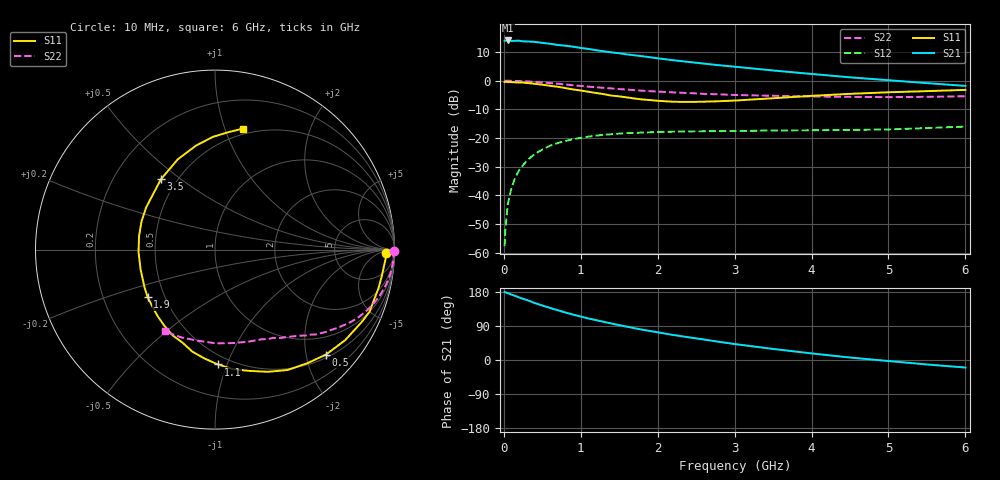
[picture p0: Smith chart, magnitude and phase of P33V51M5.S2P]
! SIEMENS Small Signal Semiconductors
! BFP181
! Si NPN RF Bipolar Junction Transistor in SOT143
! VCE = 3.5 V  IC = 1.5 mA
! Common Emitter S-Parameters:  March  1996
# GHz  S  MA  R  50
!  f  S11  S21  S12  S22
! GHz  MAG  ANG  MAG  ANG  MAG  ANG  MAG  ANG
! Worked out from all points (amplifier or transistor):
!   36 points, 10 MHz to 6 GHz, reference 50 ohm
!   highest |S21| = 14.0 dB at 50 MHz (marker M1)
!   |S21| within 3 dB of that: start of sweep to 1.109 GHz
!   unconditionally stable (mu >= 1): 2.733 GHz to end of sweep
!   at 250 MHz: K = 0.10, MSG = 21.6 dB, |S12| = -29.4 dB
!   at 1.4 GHz: K = 0.57, MSG = 14.3 dB, |S12| = -18.7 dB
!   at 6 GHz: K = 1.20, MAG = 4.4 dB, |S12| = -16.0 dB
!   S11 on the Smith chart (normalised r, x): 10 MHz: 36, -13; 500 MHz: 0.57, -2.40; 1.1 GHz: 0.43, -0.93; 1.9 GHz: 0.40, -0.27; 3.5 GHz: 0.41, +0.42; 6 GHz: 0.45, +1.15
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0.01  0.9514 -1.0  4.977 179.5  0.0013 81.9  0.9982 -0.3
0.02  0.9545 -2.0  4.986 179.0  0.0025 89.8  0.9978 -0.8
0.05  0.9488 -4.3  5.03 176.3  0.0069 91.1  0.9951 -2.0
0.1  0.941 -9.0  4.934 172.7  0.0136 82.5  0.9943 -4.1
0.2  0.9292 -17.6  4.968 165.0  0.0275 79.3  0.9856 -8.1
0.4  0.8836 -34.8  4.758 150.5  0.0526 68.3  0.9532 -15.7
0.5  0.8511 -43.4  4.569 143.6  0.0629 63.2  0.9317 -19.1
0.6  0.8158 -50.9  4.405 137.5  0.0732 58.3  0.9083 -22.3
0.8  0.7425 -66.5  4.073 125.3  0.0889 50.5  0.8599 -27.8
0.9  0.7037 -73.9  3.916 119.8  0.0955 46.6  0.8336 -30.3
1.1  0.6403 -88.5  3.578 109.5  0.1058 40.4  0.7874 -34.6
1.3  0.5825 -102.5  3.251 100.6  0.1138 34.8  0.7499 -38.4
1.5  0.5332 -116.2  3.009 91.9  0.1195 30.2  0.7135 -41.6
1.7  0.4887 -131.1  2.771 83.9  0.1227 26.7  0.6824 -44.6
1.9  0.4595 -144.8  2.566 76.5  0.1259 23.3  0.6557 -47.4
2.2  0.4292 -165.1  2.277 66.1  0.129 19.7  0.625 -51.4
2.8  0.4386 159.0  1.858 47.9  0.1322 14.1  0.5779 -59.6
3.5  0.4942 127.6  1.507 29.2  0.1355 10.5  0.5454 -70.2
4  0.544 112.4  1.31 17.4  0.1365 8.5  0.5302 -79.3
4.5  0.5892 100.3  1.144 6.5  0.1384 7.4  0.5224 -89.4
5.5  0.6576 83.7  0.907 -11.8  0.1492 7.7  0.5235 -110.6
6  0.691 77.1  0.811 -19.9  0.1583 6.8  0.5349 -121.5
